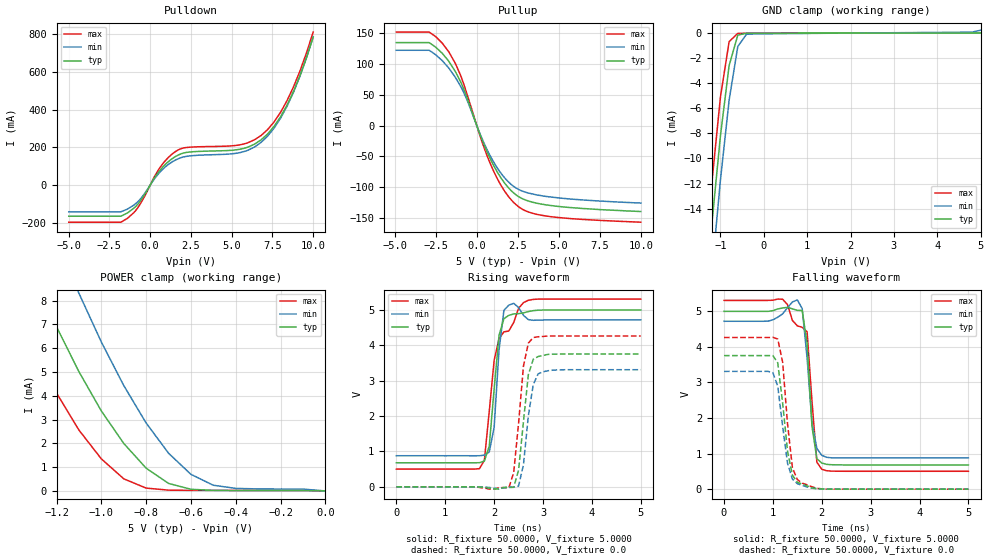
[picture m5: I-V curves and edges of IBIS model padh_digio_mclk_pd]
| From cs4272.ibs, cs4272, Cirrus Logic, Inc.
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|   Model mclkp
[Model]  padh_digio_mclk_pd
Model_type I/O
Polarity   Non-Inverting
Enable   Active-High
Vinl =   0.8000V
Vinh =   2.0000V
C_comp   5.0000pF   5.0000pF   5.0000pF
[Temperature Range]   25.0000   85.0000   -40.0000
[Voltage Range]   5.0000V   4.5000V   5.5000V
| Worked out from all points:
|   slope of the pulldown table from 0 to 0.75 V, typ, clamps not added: 8.05 ohm
|   slope of the pullup table from 0 to 0.75 V, typ, clamps not added: 15.1 ohm
|   GND clamp passes 1 mA (typ) near -0.67 V on its own axis
|   POWER clamp passes 1 mA (typ) near -0.80 V on its own axis
|   rising waveform, R_fixture 50.0000, V_fixture 5.0000: 20-80 % time 166ps typ, 112ps min, 331ps max; typ from 0.681 V to 5 V
|   rising waveform, R_fixture 50.0000, V_fixture 0.0: 20-80 % time 167ps typ, 170ps min, 167ps max; typ from 0 V to 3.75 V
|   falling waveform, R_fixture 50.0000, V_fixture 5.0000: 20-80 % time 128ps typ, 150ps min, 155ps max; typ from 5 V to 0.681 V
|   falling waveform, R_fixture 50.0000, V_fixture 0.0: 20-80 % time 199ps typ, 193ps min, 170ps max; typ from 3.75 V to 0 V
[Pulldown]
|Voltage   I(typ)   I(min)   I(max)
-5V       -165mA     -141.7mA   -196.7mA
-1.8V     -165mA     -141.7mA   -196.7mA
-900mV    -114.3mA   -99.02mA   -135.8mA
600mV     78.02mA    68.62mA    92.47mA
1.6V      153.4mA    134.6mA    180.1mA
2.4V      174.7mA    154mA      200.3mA
5.5V      189.7mA    171.8mA    213.1mA
6.8V      239mA      225.7mA    262.3mA
7.6V      310.8mA    301.3mA    334.1mA
8.4V      424mA      418.1mA    447.7mA
9.2V      581.8mA    579.1mA    606.4mA
10V       784.4mA    784mA      810.2mA
[Pullup]
|Voltage   I(typ)   I(min)   I(max)
-4.9V     134.5mA    122.1mA    151.6mA
-2.9V     134.5mA    122.1mA    151.6mA
-2.1V     117.1mA    105.2mA    133.6mA
-1.7V     104.1mA    93.09mA    119.4mA
-900mV    65.98mA    59.33mA    75.33mA
300mV     -21.63mA   -19.83mA   -24.78mA
900mV     -58.13mA   -53.14mA   -66.4mA
1.7V      -93.45mA   -84.92mA   -106.6mA
2.5V      -114.5mA   -103mA     -130.8mA
3.2V      -123mA     -109.9mA   -140.8mA
4.5V      -129.8mA   -116mA     -147.9mA
10V       -139.6mA   -125.8mA   -156.9mA
[GND_clamp]
|Voltage   I(typ)   I(min)   I(max)
-5V       -173.1mA   -172.4mA   -178.7mA
-1.4V     -23.3mA    -27.4mA    -20.12mA
-1.2V     -15.29mA   -19.22mA   -12mA
-1V       -8.186mA   -11.72mA   -5.097mA
-800mV    -2.583mA   -5.352mA   -673.4uA
-600mV    -152uA     -1.063mA   -11.24uA
-400mV    -4.543uA   -85.79uA   -4.673uA
4.8V      16.85uA    84.45uA    22.7uA
5V        16.85uA    238.4uA    22.7uA
[POWER_clamp]
|Voltage   I(typ)   I(min)   I(max)
-5V       117.7mA    125.3mA    114.4mA
-1.5V     13.66mA    18.12mA    10.24mA
-1.4V     11.25mA    15.47mA    7.995mA
-1.3V     8.988mA    12.94mA    5.941mA
-1.2V     6.901mA    10.54mA    4.116mA
-1.1V     5.014mA    8.31mA     2.559mA
-900mV    1.998mA    4.432mA    509.9uA
-800mV    956.1uA    2.856mA    118.5uA
-700mV    315.8uA    1.586mA    32.22uA
-600mV    68.65uA    695.9uA    23.28uA
-400mV    17.18uA    106.2uA    22.73uA
0V        0A         0A         0A
[Ramp]
| variable   typ   min   max
dV/dt_r  2.2530/0.1666n   1.9014/0.2064n   2.6238/0.1458n
dV/dt_f  2.5910/0.1131n   2.2349/0.1357n   NA
R_load = 50.0000
[Rising Waveform]
R_fixture= 50.0000
V_fixture= 5.0000
V_fixture_min= 5.5000
V_fixture_max= 4.5000
|time   V(typ)   V(min)   V(max)
0s        680.7mV    879.6mV    503mV
1.7ns     682.3mV    879.6mV    514.5mV
1.8ns     729.6mV    895.7mV    748.3mV
1.9ns     1.149V     983.5mV    2.132V
2ns       2.762V     1.679V     3.575V
2.1ns     4.283V     3.864V     4.186V
2.2ns     4.753V     4.989V     4.38V
2.3ns     4.847V     5.135V     4.405V
2.7ns     4.955V     4.727V     5.274V
5ns       4.999V     4.72V      5.307V
[Rising Waveform]
R_fixture= 50.0000
V_fixture= 0.0
|time   V(typ)   V(min)   V(max)
0s        0V         315.2uV    0V
2.3ns     -17.74mV   -6.679mV   -27.72mV
2.4ns     -12.89mV   -11.51mV   399.6mV
2.5ns     471.9mV    23.45mV    1.799V
2.6ns     1.846V     624.9mV    3.413V
2.7ns     3.171V     2.005V     4.062V
2.8ns     3.607V     2.889V     4.221V
2.9ns     3.683V     3.194V     4.242V
3ns       3.714V     3.253V     4.252V
5ns       3.755V     3.311V     4.264V
[Falling Waveform]
R_fixture= 50.0000
V_fixture= 5.0000
V_fixture_min= 5.5000
V_fixture_max= 4.5000
|time   V(typ)   V(min)   V(max)
0s        4.999V     4.72V      5.307V
900ps     4.999V     4.724V     5.307V
1.2ns     5.093V     4.928V     5.34V
1.5ns     5.027V     5.321V     4.592V
1.6ns     5.023V     5.077V     4.549V
1.7ns     4.098V     3.69V      4.426V
1.8ns     1.764V     1.869V     2.471V
1.9ns     856.6mV    1.145V     759.3mV
2ns       734.6mV    950.6mV    559.8mV
5ns       680.7mV    879.3mV    503mV
[Falling Waveform]
R_fixture= 50.0000
V_fixture= 0.0
|time   V(typ)   V(min)   V(max)
0s        3.755V     3.31V      4.264V
900ps     3.756V     3.312V     4.264V
1ns       3.753V     3.273V     4.268V
1.1ns     3.549V     2.893V     4.219V
1.2ns     2.418V     1.767V     3.568V
1.3ns     1.066V     725.9mV    1.837V
1.4ns     392.2mV    283.2mV    598.5mV
1.6ns     143.9mV    105.3mV    167.4mV
2.1ns     2.148mV    1.015mV    2.041mV
5ns       2.649uV    0V         878.2nV
